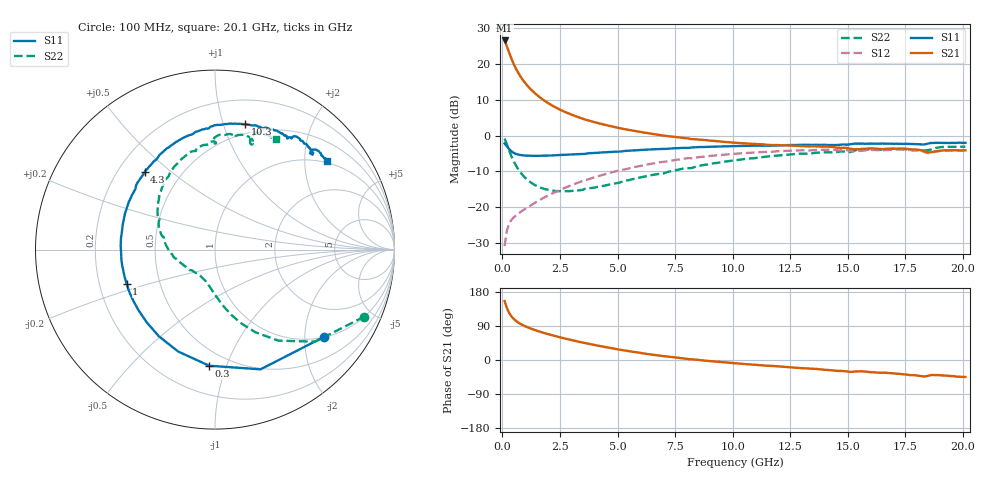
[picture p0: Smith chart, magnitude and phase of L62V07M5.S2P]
!  Infineon Technologies AG
! BFR380L3 , PF131585-7, No.6, Th 09.10.01, soldered on pcb-board, measured with PP GSG850
!  Vce=2.0 V,  Ic=7.5 mA
! Common Emitter S-Parameters:  15. November 2001
#  GHz  S  MA  R  50
! f  S11  S21  S12  S22
! GHz  Mag  Ang  Mag  Ang  Mag  Ang  Mag  Ang
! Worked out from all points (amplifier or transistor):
!   201 points, 100 MHz to 20.1 GHz, reference 50 ohm
!   highest |S21| = 26.7 dB at 100 MHz (marker M1)
!   |S21| within 3 dB of that: start of sweep to 273.5 MHz
!   unconditionally stable (mu >= 1): 1.966 GHz to 4.742 GHz
!   at 3.4 GHz: K = 1.04, MAG = 7.7 dB, |S12| = -12.9 dB
!   at 10.1 GHz: K = 0.95, MSG = 1.5 dB, |S12| = -5.1 dB
!   at 20.1 GHz: K = 0.99, MSG = 0.0 dB, |S12| = -4.1 dB
!   S11 on the Smith chart (normalised r, x): 100 MHz: 1.01, -2.48; 300 MHz: 0.39, -0.87; 1 GHz: 0.32, -0.17; 4.3 GHz: 0.31, +0.41; 10.3 GHz: 0.41, +1.19; 20.1 GHz: 0.95, +2.56
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0.1  0.7772 -38.8  21.51 155.6  0.02855 70.1  0.9112 -24.2
0.2  0.7137 -69.2  17.72 136.8  0.04741 58.4  0.7577 -42.6
0.3  0.6478 -92.9  14.41 124.0  0.05911 51.3  0.6179 -55.2
0.4  0.6036 -109.9  11.88 114.9  0.06664 47.4  0.5124 -64.0
0.5  0.5754 -122.9  9.982 108.1  0.07221 46.0  0.436 -70.4
0.6  0.5559 -133.2  8.577 102.9  0.07701 45.5  0.3795 -75.5
0.7  0.5441 -141.5  7.505 98.5  0.08158 45.8  0.3362 -79.6
0.8  0.5368 -148.3  6.655 94.9  0.0861 46.3  0.3034 -83.1
1  0.5278 -158.9  5.428 88.8  0.09517 47.8  0.2566 -89.1
1.2  0.5245 -167.2  4.578 83.8  0.1047 49.3  0.2264 -94.2
1.4  0.5243 -173.9  3.964 79.4  0.1146 50.7  0.2054 -98.9
1.9  0.5278 172.8  2.984 69.8  0.1411 52.8  0.1779 -109.5
2.6  0.5401 158.3  2.241 58.5  0.1803 53.4  0.1673 -123.6
3.5  0.5565 143.4  1.725 45.8  0.2337 51.5  0.1755 -139.3
4.3  0.583 132.3  1.461 36.1  0.2807 48.5  0.1965 -154.6
5.2  0.6054 121.6  1.254 26.1  0.3328 43.3  0.2283 -167.8
6.8  0.6513 103.9  1.028 11.6  0.4234 33.9  0.2922 167.5
10.1  0.7161 77.9  0.7976 -8.6  0.559 12.2  0.4548 130.4
10.3  0.7194 76.4  0.7895 -9.4  0.5653 11.0  0.4623 128.2
13.5  0.7452 59.9  0.7136 -23.2  0.6292 -9.2  0.5713 100.2
16.8  0.7725 47.8  0.6584 -34.2  0.6324 -25.5  0.6537 77.9
20.1  0.7958 38.4  0.6267 -44.8  0.6237 -39.2  0.7032 61.3
